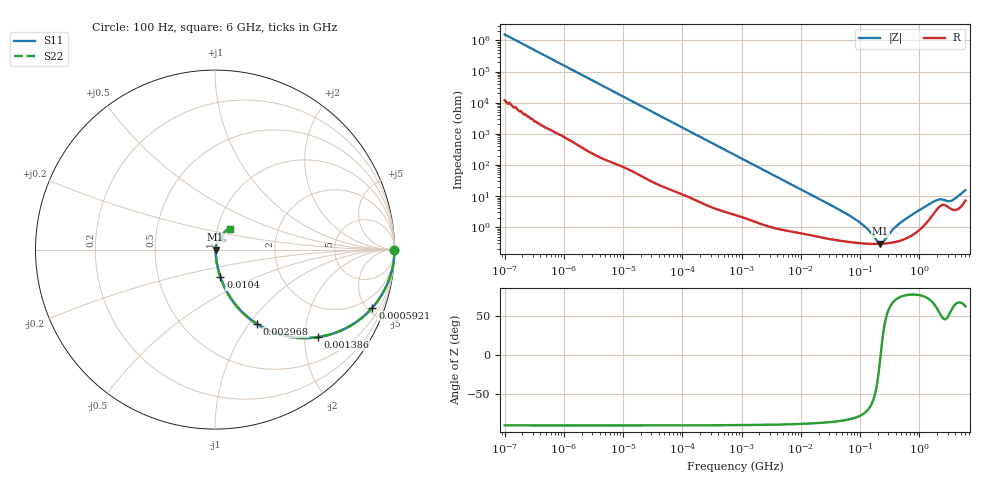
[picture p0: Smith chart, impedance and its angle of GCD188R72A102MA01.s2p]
!Murata Part Number: GCD188R72A102MA01
!These Parameters are Measured in Series Mode Connection
!Data Generated on Jan 08, 2026
!  o--ll--o
!Port1  Port2
!  o------o
!Operation Temp=25[degC], DC Bias Voltage=0[V]
!Freq. Start=100[Hz] Stop=6[GHz] 401[Steps]
# Hz S RI R 50
!Freq.(Hz) S11(Real) S11(Imag) S21(Real) S21(Imag) S12(Real) S12(Imag) S22(Real) S22(Imag)
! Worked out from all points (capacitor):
!   401 points, 100 Hz to 6 GHz, reference 50 ohm
!   read as one part in series: C = 1.02 nF near 109 Hz
!   lowest |Z| = 294 mohm at 218.4 MHz (marker M1)
!   series resonance near 222.2 MHz, so ESL is about 500 pH
!   S11 on the Smith chart (normalised r, x): 100 Hz: open; 592.1 kHz: 1.06, -5.41; 1.386 MHz: 1.03, -2.32; 2.968 MHz: 1.02, -1.09; 10.4 MHz: 1.01, -0.31; 6 GHz: 1.14, +0.27
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100  1 -6.45e-05  5e-07 6.45e-05  5e-07 6.45e-05  1 -6.45e-05
164  1 -0.000105  7e-07 0.000105  7e-07 0.000105  1 -0.000105
2008  1 -0.00128  7.6e-06 0.00128  7.6e-06 0.00128  1 -0.00128
40335  0.9992 -0.0255  0.000797 0.0255  0.000797 0.0255  0.9992 -0.0255
184852  0.9858 -0.1143  0.0142 0.1143  0.0142 0.1143  0.9858 -0.1143
592111  0.877 -0.3231  0.123 0.3231  0.123 0.3231  0.877 -0.3231
774597  0.8078 -0.388  0.1922 0.388  0.1922 0.388  0.8078 -0.388
1386327  0.5734 -0.4873  0.4266 0.4873  0.4266 0.4873  0.5734 -0.4873
2967816  0.2337 -0.4138  0.7663 0.4138  0.7663 0.4138  0.2337 -0.4138
5079039  0.0988 -0.286  0.9012 0.286  0.9012 0.286  0.0988 -0.286
1.039699e7  0.03 -0.1518  0.97 0.1518  0.97 0.1518  0.03 -0.1518
1.555665e7  0.0162 -0.1034  0.9838 0.1034  0.9838 0.1034  0.0162 -0.1034
8.918374e7  0.00338 -0.016  0.9966 0.016  0.9966 0.016  0.00338 -0.016
1.334425e8  0.00301 -0.00822  0.997 0.00822  0.997 0.00822  0.00301 -0.00822
2.183701e8  0.00292 -0.000269  0.9971 0.000269  0.9971 0.000269  0.00292 -0.000269
2.497637e8  0.00296 0.00182  0.997 -0.00182  0.997 -0.00182  0.00296 0.00182
3.124326e8  0.00312 0.00541  0.9969 -0.00541  0.9969 -0.00541  0.00312 0.00541
5.346885e8  0.0042 0.0156  0.9958 -0.0156  0.9958 -0.0156  0.0042 0.0156
1.565993e9  0.0229 0.0531  0.9771 -0.0531  0.9771 -0.0531  0.0229 0.0531
2.142435e9  0.0456 0.0584  0.9544 -0.0584  0.9544 -0.0584  0.0456 0.0584
3.505958e9  0.0397 0.0561  0.9603 -0.0561  0.9603 -0.0561  0.0397 0.0561
6e9  0.0816 0.1175  0.9184 -0.1175  0.9184 -0.1175  0.0816 0.1175
